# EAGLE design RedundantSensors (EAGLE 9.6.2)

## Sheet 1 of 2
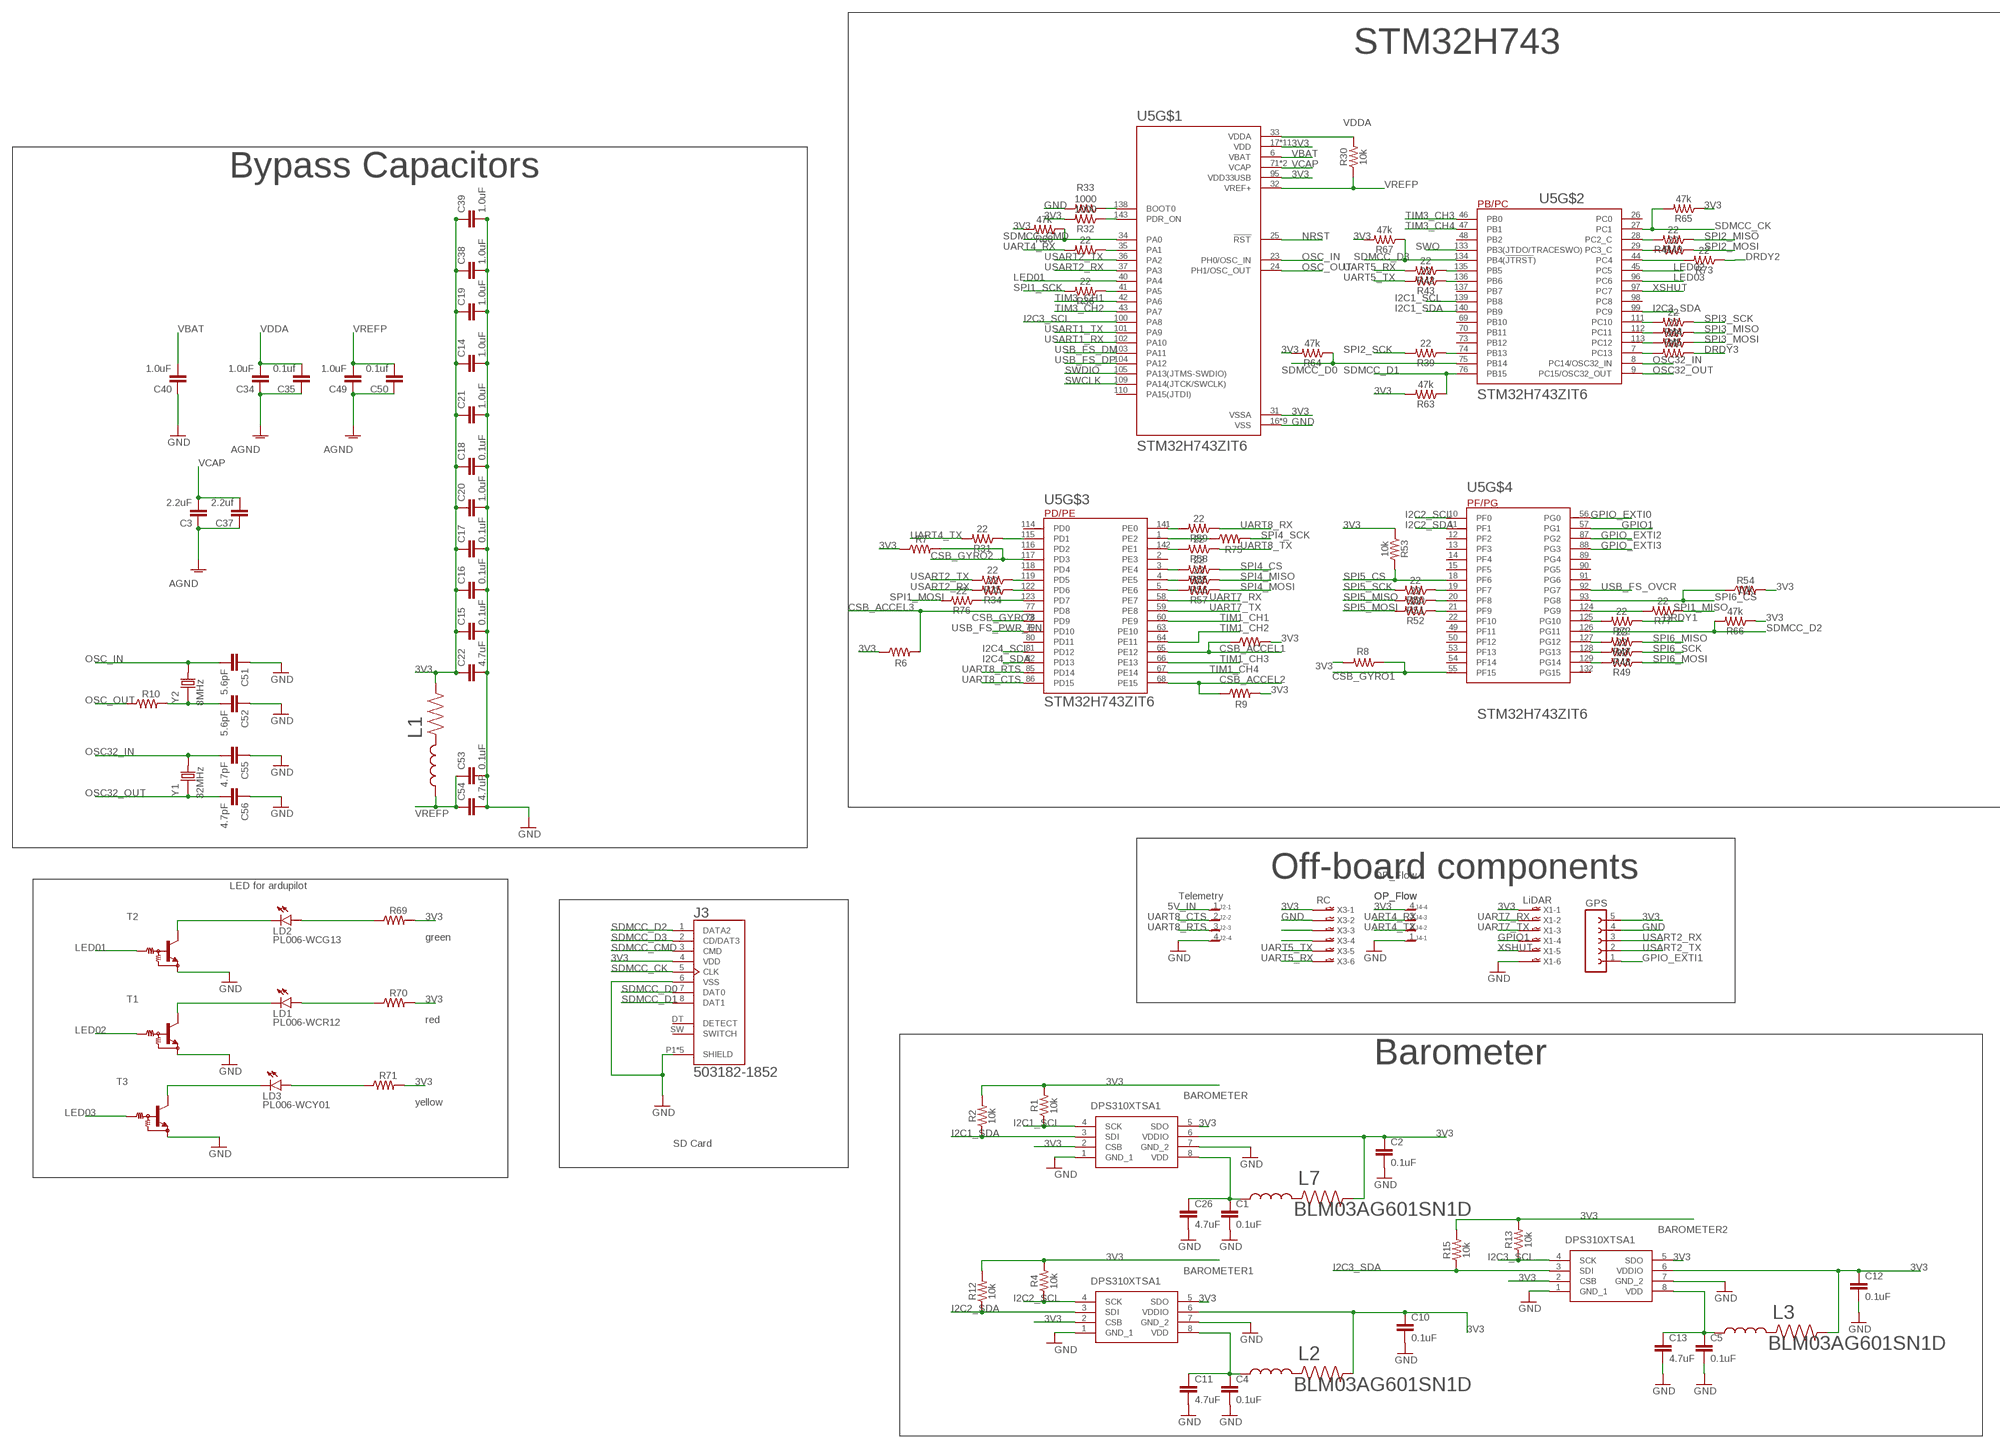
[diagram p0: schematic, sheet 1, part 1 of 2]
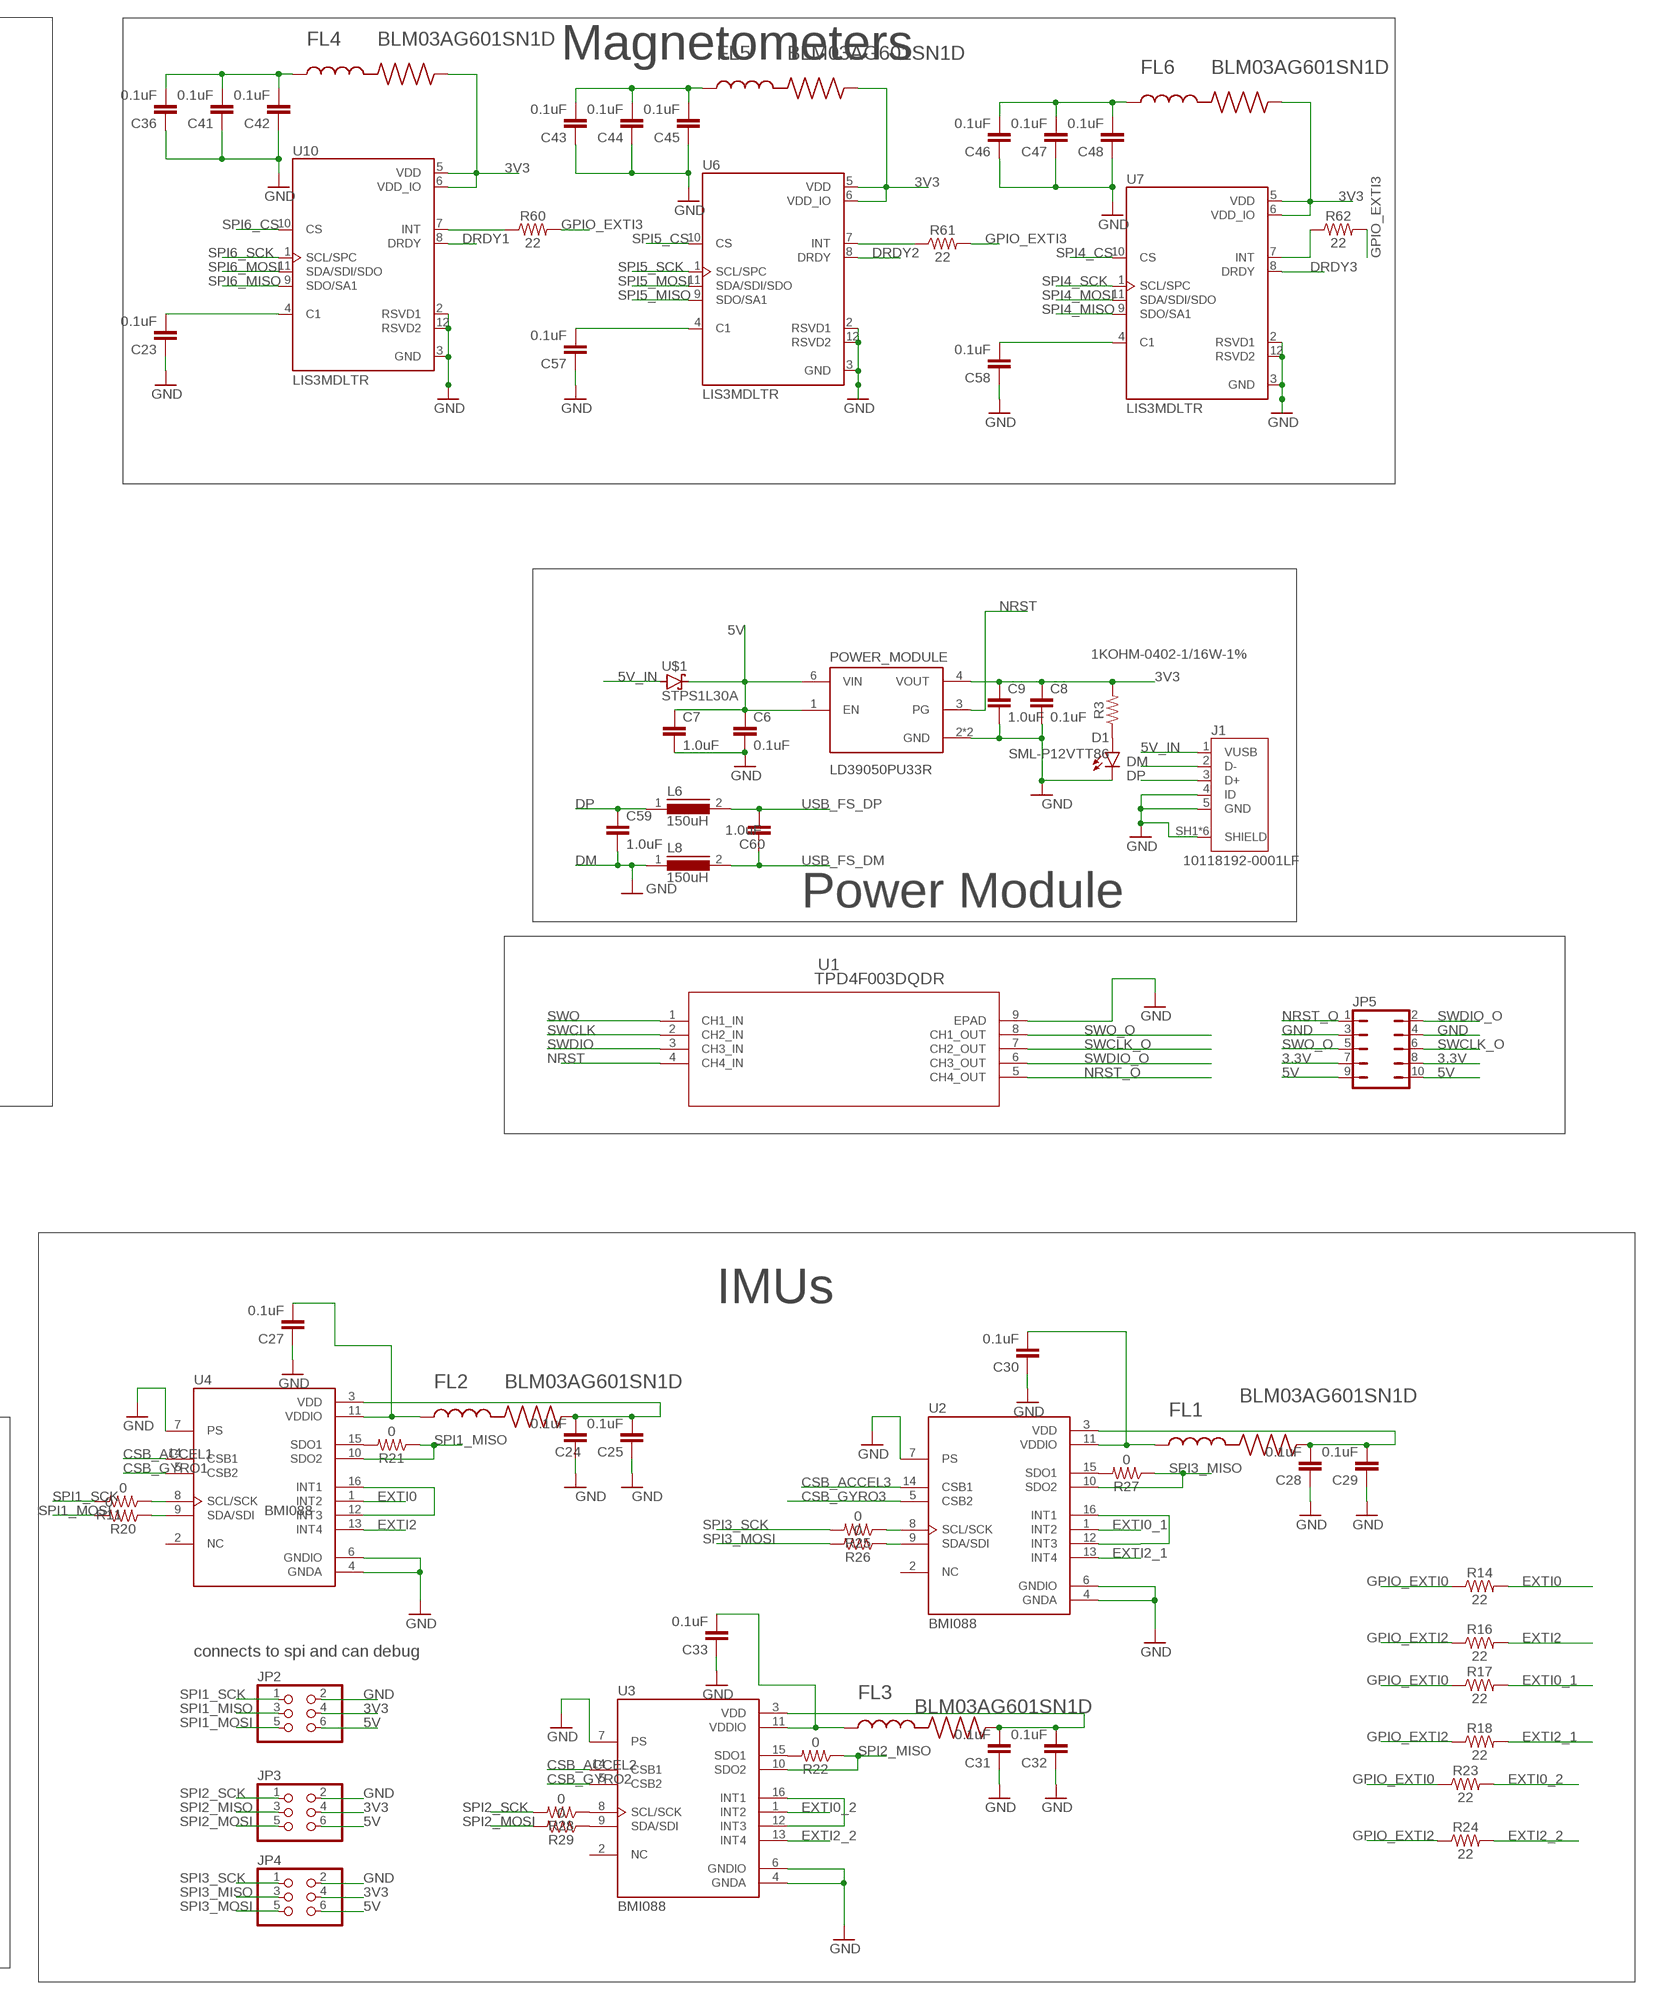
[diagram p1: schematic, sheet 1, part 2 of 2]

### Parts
BAROMETER  DPS310XTSA1  [DPS310XTSA1]
BAROMETER1  DPS310XTSA1  [DPS310XTSA1]
BAROMETER2  DPS310XTSA1  [DPS310XTSA1]
C1  0.1uF  0.1UF-0402-6.3V-10%-X7R  [0402]
C2  0.1uF  0.1UF-0402-6.3V-10%-X7R  [0402]
C3  2.2uF  1.0UF-0805-25V-10%  [0805]
C4  0.1uF  0.1UF-0402-6.3V-10%-X7R  [0402]
C5  0.1uF  0.1UF-0402-6.3V-10%-X7R  [0402]
C6  0.1uF  0.1UF-0402-6.3V-10%-X7R  [0402]
C7  1.0uF  1.0UF-0402-16V-10%  [0402]
C8  0.1uF  0.1UF-0402-6.3V-10%-X7R  [0402]
C9  1.0uF  1.0UF-0402-16V-10%  [0402]
C10  0.1uF  0.1UF-0402-6.3V-10%-X7R  [0402]
C11  4.7uF  4.7UF0603  [0603]
C12  0.1uF  0.1UF-0402-6.3V-10%-X7R  [0402]
C13  4.7uF  4.7UF0603  [0603]
C14  1.0uF  1.0UF-0805-25V-10%  [0805]
C15  0.1uF  0.1UF-0603-25V-5%  [0603]
C16  0.1uF  0.1UF-0603-25V-5%  [0603]
C17  0.1uF  0.1UF-0603-25V-5%  [0603]
C18  0.1uF  0.1UF-0603-25V-5%  [0603]
C19  1.0uF  1.0UF-0805-25V-10%  [0805]
C20  1.0uF  1.0UF-0805-25V-10%  [0805]
C21  1.0uF  1.0UF-0805-25V-10%  [0805]
C22  4.7uF  4.7UF0603  [0603]
C23  0.1uF  0.1UF-0603-25V-5%  [0603]
C24  0.1uF  0.1UF-0603-25V-5%  [0603]
C25  0.1uF  0.1UF-0603-25V-5%  [0603]
C26  4.7uF  4.7UF0603  [0603]
C27  0.1uF  0.1UF-0603-25V-5%  [0603]
C28  0.1uF  0.1UF-0603-25V-5%  [0603]
C29  0.1uF  0.1UF-0603-25V-5%  [0603]
C30  0.1uF  0.1UF-0603-25V-5%  [0603]
C31  0.1uF  0.1UF-0603-25V-5%  [0603]
C32  0.1uF  0.1UF-0603-25V-5%  [0603]
C33  0.1uF  0.1UF-0603-25V-5%  [0603]
C34  1.0uF  1.0UF-0805-25V-10%  [0805]
C35  0.1uf  1.0UF-0805-25V-10%  [0805]
C36  0.1uF  0.1UF-0603-25V-5%  [0603]
C37  2.2uf  1.0UF-0805-25V-10%  [0805]
C38  1.0uF  1.0UF-0805-25V-10%  [0805]
C39  1.0uF  1.0UF-0805-25V-10%  [0805]
C40  1.0uF  1.0UF-0805-25V-10%  [0805]
C41  0.1uF  0.1UF-0603-25V-5%  [0603]
C42  0.1uF  0.1UF-0603-25V-5%  [0603]
C43  0.1uF  0.1UF-0603-25V-5%  [0603]
C44  0.1uF  0.1UF-0603-25V-5%  [0603]
C45  0.1uF  0.1UF-0603-25V-5%  [0603]
C46  0.1uF  0.1UF-0603-25V-5%  [0603]
C47  0.1uF  0.1UF-0603-25V-5%  [0603]
C48  0.1uF  0.1UF-0603-25V-5%  [0603]
C49  1.0uF  1.0UF-0805-25V-10%  [0805]
C50  0.1uf  1.0UF-0805-25V-10%  [0805]
C51  5.6pF  1.0UF-0805-25V-10%  [0805]
C52  5.6pF  1.0UF-0805-25V-10%  [0805]
C53  0.1uF  0.1UF-0603-25V-5%  [0603]
C54  4.7uF  4.7UF0603  [0603]
C55  4.7pF  1.0UF-0805-25V-10%  [0805]
C56  4.7pF  1.0UF-0805-25V-10%  [0805]
C57  0.1uF  0.1UF-0603-25V-5%  [0603]
C58  0.1uF  0.1UF-0603-25V-5%  [0603]
C59  1.0uF  1.0UF-0402-16V-10%  [0402]
C60  1.0uF  1.0UF-0402-16V-10%  [0402]
D1  SML-P12VTT86  [LED_SML-P11UTT86R]
FL1  BLM03AG601SN1D  [BEADC0603X33N]
FL2  BLM03AG601SN1D  [BEADC0603X33N]
FL3  BLM03AG601SN1D  [BEADC0603X33N]
FL4  BLM03AG601SN1D  [BEADC0603X33N]
FL5  BLM03AG601SN1D  [BEADC0603X33N]
FL6  BLM03AG601SN1D  [BEADC0603X33N]
GPS  FE05-1  [FE05-1]
J1  10118192-0001LF  [AMPHENOL_10118192-0001LF]
J2  JST-SH-4_SMT_V  [BM04B-SRSS-TB]
J3  503182-1852  [MOLEX_503182-1852]
J4  JST-SH-4_SMT_V  [BM04B-SRSS-TB]
JP2  PINHD-2X3  [2X03]
JP3  PINHD-2X3  [2X03]
JP4  PINHD-2X3  [2X03]
JP5  JP5Q  [JP5Q]
L1  BLM03AG601SN1D  [BEADC0603X33N]
L2  BLM03AG601SN1D  [BEADC0603X33N]
L3  BLM03AG601SN1D  [BEADC0603X33N]
L6  150uH  MICC10  [MICC10]
L7  BLM03AG601SN1D  [BEADC0603X33N]
L8  150uH  MICC10  [MICC10]
LD1  PL006-WCR12  [SOT23]
LD2  PL006-WCG13  PL006-WCR12  [SOT23]
LD3  PL006-WCY01  PL006-WCR12  [SOT23]
POWER_MODULE  LD39050PU33R  [SON95P300X300X100-7N]
R1  10k  10KOHM-0402-1/16W-1%  [0402]
R2  10k  10KOHM-0402-1/16W-1%  [0402]
R3  1KOHM-0402-1/16W-1%  [0402]
R4  10k  10KOHM-0402-1/16W-1%  [0402]
R5  22  10KOHM-0402-1/16W-1%  [0402]
R6  10k  RT0402FRE07220RL  [RESC1005X35N]
R7  10k  RT0402FRE07220RL  [RESC1005X35N]
R8  10k  RT0402FRE07220RL  [RESC1005X35N]
R9  10k  RT0402FRE07220RL  [RESC1005X35N]
R10  220  RT0402FRE07220RL  [RESC1005X35N]
R11  0  10KOHM-0402-1/16W-1%  [0402]
R12  10k  10KOHM-0402-1/16W-1%  [0402]
R13  10k  10KOHM-0402-1/16W-1%  [0402]
R14  22  22OHM-0402-1/10W-1%  [0402]
R15  10k  10KOHM-0402-1/16W-1%  [0402]
R16  22  22OHM-0402-1/10W-1%  [0402]
R17  22  22OHM-0402-1/10W-1%  [0402]
R18  22  22OHM-0402-1/10W-1%  [0402]
R19  10k  RT0402FRE07220RL  [RESC1005X35N]
R20  0  10KOHM-0402-1/16W-1%  [0402]
R21  0  10KOHM-0402-1/16W-1%  [0402]
R22  0  10KOHM-0402-1/16W-1%  [0402]
R23  22  22OHM-0402-1/10W-1%  [0402]
R24  22  22OHM-0402-1/10W-1%  [0402]
R25  0  10KOHM-0402-1/16W-1%  [0402]
R26  0  10KOHM-0402-1/16W-1%  [0402]
R27  0  10KOHM-0402-1/16W-1%  [0402]
R28  0  10KOHM-0402-1/16W-1%  [0402]
R29  0  10KOHM-0402-1/16W-1%  [0402]
R30  10k  10KOHM-0402-1/16W-1%  [0402]
R31  22  10KOHM-0402-1/16W-1%  [0402]
R32  1000  10KOHM-0402-1/16W-1%  [0402]
R33  1000  10KOHM-0402-1/16W-1%  [0402]
R34  22  10KOHM-0402-1/16W-1%  [0402]
R35  22  10KOHM-0402-1/16W-1%  [0402]
R36  22  10KOHM-0402-1/16W-1%  [0402]
R39  22  10KOHM-0402-1/16W-1%  [0402]
R40  22  10KOHM-0402-1/16W-1%  [0402]
R41  22  10KOHM-0402-1/16W-1%  [0402]
R42  22  10KOHM-0402-1/16W-1%  [0402]
R43  22  10KOHM-0402-1/16W-1%  [0402]
R44  22  10KOHM-0402-1/16W-1%  [0402]
R45  22  10KOHM-0402-1/16W-1%  [0402]
R46  22  10KOHM-0402-1/16W-1%  [0402]
R47  22  10KOHM-0402-1/16W-1%  [0402]
R48  22  10KOHM-0402-1/16W-1%  [0402]
R49  22  10KOHM-0402-1/16W-1%  [0402]
R50  22  10KOHM-0402-1/16W-1%  [0402]
R51  22  10KOHM-0402-1/16W-1%  [0402]
R52  22  10KOHM-0402-1/16W-1%  [0402]
R53  10k  10KOHM-0402-1/16W-1%  [0402]
R54  10k  10KOHM-0402-1/16W-1%  [0402]
R55  22  10KOHM-0402-1/16W-1%  [0402]
R56  22  10KOHM-0402-1/16W-1%  [0402]
R57  22  10KOHM-0402-1/16W-1%  [0402]
R58  22  10KOHM-0402-1/16W-1%  [0402]
R59  22  10KOHM-0402-1/16W-1%  [0402]
R60  22  22OHM-0402-1/10W-1%  [0402]
R61  22  22OHM-0402-1/10W-1%  [0402]
R62  22  22OHM-0402-1/10W-1%  [0402]
R63  47k  10KOHM-0402-1/16W-1%  [0402]
R64  47k  10KOHM-0402-1/16W-1%  [0402]
R65  47k  10KOHM-0402-1/16W-1%  [0402]
R66  47k  10KOHM-0402-1/16W-1%  [0402]
R67  47k  10KOHM-0402-1/16W-1%  [0402]
R68  47k  10KOHM-0402-1/16W-1%  [0402]
R69  270  RT0402FRE07220RL  [RESC1005X35N]
R70  270  RT0402FRE07220RL  [RESC1005X35N]
R71  270  RT0402FRE07220RL  [RESC1005X35N]
R72  22  10KOHM-0402-1/16W-1%  [0402]
R73  22  10KOHM-0402-1/16W-1%  [0402]
R74  22  10KOHM-0402-1/16W-1%  [0402]
R75  10k  RT0402FRE07220RL  [RESC1005X35N]
R76  22  10KOHM-0402-1/16W-1%  [0402]
R77  22  10KOHM-0402-1/16W-1%  [0402]
T1  MUN2213T1-NPN_DRIVER-SC59-BEC  [SC59-BEC]
T2  MUN2213T1-NPN_DRIVER-SC59-BEC  [SC59-BEC]
T3  MUN2213T1-NPN_DRIVER-SC59-BEC  [SC59-BEC]
U1  TPD4F003DQDR  [DQD8_1P2X0P4]
U2  BMI088  [PQFN50P450X300X100-16N]
U3  BMI088  [PQFN50P450X300X100-16N]
U4  BMI088  [PQFN50P450X300X100-16N]
U5  STM32H743ZIT6  [QFP50P2200X2200X160-144N]
U6  LIS3MDLTR  [XDCR_LIS3MDLTR]
U7  LIS3MDLTR  [XDCR_LIS3MDLTR]
U10  LIS3MDLTR  [XDCR_LIS3MDLTR]
U$1  STPS1L30A  [DIOM5226X223N]
X1  LiDAR  06FLZ-SM1  [6FLZ-SM]
X3  RC  06FLZ-SM1  [6FLZ-SM]
Y1  32MHz  ABLS-8.000MHZ-B2-T  [XTAL_ABLS-8.000MHZ-B2-T]
Y2  8MHz  ABLS-8.000MHZ-B2-T  [XTAL_ABLS-8.000MHZ-B2-T]

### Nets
3.3V: JP5.7 JP5.8
3V2: C28.2 C29.2 FL1.2 U2.3(VDD)
3V3: BAROMETER1.2(CSB) BAROMETER1.5(SDO) BAROMETER1.6(VDDIO) BAROMETER2.2(CSB) BAROMETER2.5(SDO) BAROMETER2.6(VDDIO) BAROMETER.2(CSB) BAROMETER.5(SDO) BAROMETER.6(VDDIO) C2.1 C8.1 C9.1 C10.1 C12.1 C14.1 C15.1 C16.1 C17.1 C18.1 C19.1 C20.1 C21.1 C22.1 C38.1 C39.1 FL4.2 FL5.2 FL6.2 GPS.5 J3.4(VDD) J4.4 JP2.4 JP3.4 JP4.4 L1.2 L2.2 L3.2 L7.2 POWER_MODULE.4(VOUT) R1.2 R2.2 R3.2 R4.2 R6.1 R7.1 R8.2 R9.2 R12.2 R13.2 R15.2 R19.2 R32.2 R53.1 R54.2 R63.2 R64.2 R65.1 R66.1 R67.2 R68.2 R69.2 R70.2 R71.2 U5.17(VDD) U5.30(VDD) U5.31(VSSA) U5.39(VDD) U5.52(VDD) U5.62(VDD) U5.72(VDD) U5.84(VDD) U5.95(VDD33USB) U5.108(VDD) U5.121(VDD) U5.131(VDD) U5.144(VDD) U6.5(VDD) U6.6(VDD_IO) U7.5(VDD) U7.6(VDD_IO) U10.5(VDD) U10.6(VDD_IO) X1.1 X3.1
3V4: C24.2 C25.2 FL2.2 U4.3(VDD)
3V5: C31.2 C32.2 FL3.2 U3.3(VDD)
5V: C6.1 C7.1 JP2.6 JP3.6 JP4.6 JP5.9 JP5.10 POWER_MODULE.1(EN) POWER_MODULE.6(VIN) U$1.1(C)
5V_IN: J1.1(VUSB) J2.1 U$1.2(A)
AGND: C3.1 C34.1 C35.1 C37.1 C49.1 C50.1
CSB_ACCEL1: R19.1 U4.14(CSB1) U5.65(PE12)
CSB_ACCEL2: R9.1 U3.14(CSB1) U5.68(PE15)
CSB_ACCEL3: R6.2 U2.14(CSB1) U5.77(PD8)
CSB_GYRO1: R8.1 U4.5(CSB2) U5.55(PF15)
CSB_GYRO2: R7.2 U3.5(CSB2) U5.117(PD3)
CSB_GYRO3: U2.5(CSB2) U5.78(PD9)
DM: C59.2 J1.2(D-) L8.1 ; supply symbol labelled GND
DP: C59.1 J1.3(D+) L6.1
DRDY1: R72.1 U10.8(DRDY)
DRDY2: R73.1 R73.2 U5.44(PC4) U6.8(DRDY)
DRDY3: R74.1 U7.8(DRDY)
EXTI0: R14.2 U4.1(INT2)
EXTI0_1: R17.2 U2.1(INT2)
EXTI0_2: R23.2 U3.1(INT2)
EXTI2: R16.2 U4.13(INT4)
EXTI2_1: R18.2 U2.13(INT4)
EXTI2_2: R24.2 U3.13(INT4)
GND: BAROMETER1.1(GND_1) BAROMETER1.7(GND_2) BAROMETER2.1(GND_1) BAROMETER2.7(GND_2) BAROMETER.1(GND_1) BAROMETER.7(GND_2) C1.2 C2.2 C4.2 C5.2 C6.2 C7.2 C8.2 C9.2 C10.2 C11.2 C12.2 C13.2 C14.2 C15.2 C16.2 C17.2 C18.2 C19.2 C20.2 C21.2 C22.2 C23.1 C24.1 C25.1 C26.2 C27.1 C28.1 C29.1 C30.1 C31.1 C32.1 C33.1 C36.1 C38.2 C39.2 C40.1 C41.1 C42.1 C43.1 C44.1 C45.1 C46.1 C47.1 C48.1 C51.1 C52.1 C53.2 C54.2 C55.1 C56.1 C57.1 C58.1 D1.C GPS.4 J1.4(ID) J1.5(GND) J1.SH1(SHIELD) J1.SH2(SHIELD) J1.SH3(SHIELD) J1.SH4(SHIELD) J1.SH5(SHIELD) J1.SH6(SHIELD) J3.6(VSS) J3.P1(SHIELD) J3.P2(SHIELD) J3.P3(SHIELD) J3.P4(SHIELD) J3.P5(SHIELD) J4.1 JP2.2 JP3.2 JP4.2 JP5.3 JP5.4 POWER_MODULE.2(GND) POWER_MODULE.7(GND) R33.2 T1.E T2.E T3.E U1.9(EPAD) U2.4(GNDA) U2.6(GNDIO) U2.7(PS) U3.4(GNDA) U3.6(GNDIO) U3.7(PS) U4.4(GNDA) U4.6(GNDIO) U4.7(PS) U5.16(VSS) U5.38(VSS) U5.51(VSS) U5.61(VSS) U5.83(VSS) U5.94(VSS) U5.107(VSS) U5.120(VSS) U5.130(VSS) U6.2(RSVD1) U6.3(GND) U6.12(RSVD2) U7.2(RSVD1) U7.3(GND) U7.12(RSVD2) U10.2(RSVD1) U10.3(GND) U10.12(RSVD2) X1.6 X3.2
GPIO1: U5.57(PG1) X1.4
GPIO_EXTI0: R14.1 R17.1 R23.1 U5.56(PG0)
GPIO_EXTI1: GPS.1
GPIO_EXTI2: R16.1 R18.1 R24.1 U5.87(PG2)
GPIO_EXTI3: R60.2 R61.2 R62.2 U5.88(PG3)
I2C1_SCL: BAROMETER.4(SCK) R1.1 U5.139(PB8)
I2C1_SDA: BAROMETER.3(SDI) R2.1 U5.140(PB9)
I2C2_SCL: BAROMETER1.4(SCK) R4.1 U5.10(PF0)
I2C2_SDA: BAROMETER1.3(SDI) R12.1 U5.11(PF1)
I2C3_SCL: BAROMETER2.4(SCK) R13.1 U5.100(PA8)
I2C3_SDA: BAROMETER2.3(SDI) R15.1 U5.99(PC9)
I2C4_SCL: U5.81(PD12)
I2C4_SDA: U5.82(PD13)
INT1: U2.12(INT3) U2.16(INT1)
LED01: T2.B U5.40(PA4)
LED02: T1.B U5.45(PC5)
LED03: T3.B U5.96(PC6)
N$1: U4.12(INT3) U4.16(INT1)
N$2: BAROMETER2.8(VDD) C5.1 C13.1 L3.1
N$3: BAROMETER1.8(VDD) C4.1 C11.1 L2.1
N$4: U3.12(INT3) U3.16(INT1)
N$5: D1.A R3.1
N$6: BAROMETER.8(VDD) C1.1 C26.1 L7.1
N$7: C52.2 R10.2 Y2.1
N$8: C27.2 FL2.1 U4.11(VDDIO)
N$9: C30.2 FL1.1 U2.11(VDDIO)
N$10: C33.2 FL3.1 U3.11(VDDIO)
N$11: C23.2 U10.4(C1)
N$12: R32.1 U5.143(PDR_ON)
N$13: R55.2 U5.3(PE4)
N$14: R56.2 U5.4(PE5)
N$15: X3.4
N$16: C36.2 C41.2 C42.2 FL4.1
N$17: C57.2 U6.4(C1)
N$18: R33.1 U5.138(BOOT0)
N$19: J2.4 ; supply symbol labelled GND
N$20: R5.1 U5.35(PA1)
N$21: R11.1 U4.8(SCL/SCK)
N$22: R20.1 U4.9(SDA/SDI)
N$23: R40.2 U5.28(PC2_C)
N$24: R21.2 U4.15(SDO1)
N$25: R22.2 U3.15(SDO1)
N$26: R25.1 U2.8(SCL/SCK)
N$27: R26.1 U2.9(SDA/SDI)
N$28: R27.2 U2.15(SDO1)
N$29: R28.1 U3.8(SCL/SCK)
N$30: R29.1 U3.9(SDA/SDI)
N$31: R34.1 U5.122(PD6)
N$32: R35.1 U5.119(PD5)
N$33: R36.1 U5.41(PA5)
N$36: R39.1 U5.74(PB13)
N$37: R41.2 U5.29(PC3_C)
N$38: R31.1 U5.115(PD1)
N$39: R42.1 U5.135(PB5)
N$40: R43.1 U5.136(PB6)
N$41: R44.2 U5.111(PC10)
N$42: R45.2 U5.112(PC11)
N$43: R46.2 U5.113(PC12)
N$44: R47.2 U5.127(PG12)
N$45: R48.2 U5.128(PG13)
N$46: R49.2 U5.129(PG14)
N$47: R50.1 U5.19(PF7)
N$48: R51.1 U5.20(PF8)
N$49: R52.1 U5.21(PF9)
N$50: R57.2 U5.5(PE6)
N$51: R58.2 U5.142(PE1)
N$52: R59.2 U5.141(PE0)
N$53: C43.2 C44.2 C45.2 FL5.1
N$54: C58.2 U7.4(C1)
N$55: C46.2 C47.2 C48.2 FL6.1
N$56: R60.1 U10.7(INT)
N$57: R61.1 U6.7(INT)
N$58: R62.1 U7.7(INT)
N$59: LD2.3(C) T2.C
N$60: LD2.1(A) R69.1
N$61: LD1.3(C) T1.C
N$62: LD1.1(A) R70.1
N$63: LD3.3(C) T3.C
N$64: LD3.1(A) R71.1
N$65: R72.2 U5.125(PG10)
N$66: R74.2 U5.7(PC13)
N$67: R75.1 U5.1(PE2)
N$68: R76.1 U5.123(PD7)
N$69: R77.2 U5.124(PG9)
NRST: POWER_MODULE.3(PG) U1.4(CH4_IN) U5.25(!RST)
NRST_O: JP5.1 U1.5(CH4_OUT)
OSC32_IN: C55.2 U5.8(PC14/OSC32_IN) Y1.2
OSC32_OUT: C56.2 U5.9(PC15/OSC32_OUT) Y1.1
OSC_IN: C51.2 U5.23(PH0/OSC_IN) Y2.2
OSC_OUT: R10.1 U5.24(PH1/OSC_OUT)
SDMCC_CK: J3.5(CLK) R65.2 U5.27(PC1)
SDMCC_CMD: J3.3(CMD) R68.1 U5.34(PA0)
SDMCC_D0: J3.7(DAT0) R64.1 U5.75(PB14)
SDMCC_D1: J3.8(DAT1) R63.1 U5.76(PB15)
SDMCC_D2: J3.1(DATA2) R66.2 U5.126(PG11)
SDMCC_D3: J3.2(CD/DAT3) R67.1 U5.134(PB4(!JTRST!))
SPI1_MISO: JP2.3 R21.1 R77.1 U4.10(SDO2)
SPI1_MOSI: JP2.5 R20.2 R76.2
SPI1_SCK: JP2.1 R11.2 R36.2
SPI2_MISO: JP3.3 R22.1 R40.1 U3.10(SDO2)
SPI2_MOSI: JP3.5 R29.2 R41.1
SPI2_SCK: JP3.1 R28.2 R39.2
SPI3_MISO: JP4.3 R27.1 R45.1 U2.10(SDO2)
SPI3_MOSI: JP4.5 R26.2 R46.1
SPI3_SCK: JP4.1 R25.2 R44.1
SPI4_CS: R55.1 U7.10(CS)
SPI4_MISO: R56.1 U7.9(SDO/SA1)
SPI4_MOSI: R57.1 U7.11(SDA/SDI/SDO)
SPI4_SCK: R75.2 U7.1(SCL/SPC)
SPI5_CS: R53.2 U5.18(PF6) U6.10(CS)
SPI5_MISO: R51.2 U6.9(SDO/SA1)
SPI5_MOSI: R52.2 U6.11(SDA/SDI/SDO)
SPI5_SCK: R50.2 U6.1(SCL/SPC)
SPI6_CS: R54.1 U5.93(PG8) U10.10(CS)
SPI6_MISO: R47.1 U10.9(SDO/SA1)
SPI6_MOSI: R49.1 U10.11(SDA/SDI/SDO)
SPI6_SCK: R48.1 U10.1(SCL/SPC)
SWCLK: U1.2(CH2_IN) U5.109(PA14(JTCK/SWCLK))
SWCLK_O: JP5.6 U1.7(CH2_OUT)
SWDIO: U1.3(CH3_IN) U5.105(PA13(JTMS-SWDIO))
SWDIO_O: JP5.2 U1.6(CH3_OUT)
SWO: U1.1(CH1_IN) U5.133(PB3(JTDO/TRACESWO))
SWO_O: JP5.5 U1.8(CH1_OUT)
TIM1_CH1: U5.60(PE9)
TIM1_CH2: U5.64(PE11)
TIM1_CH3: U5.66(PE13)
TIM1_CH4: U5.67(PE14)
TIM3_CH1: U5.42(PA6)
TIM3_CH2: U5.43(PA7)
TIM3_CH3: U5.46(PB0)
TIM3_CH4: U5.47(PB1)
UART4_RX: J4.3 R5.2
UART4_TX: J4.2 R31.2
UART5_RX: R42.2 X3.3 X3.6
UART5_TX: R43.2 X3.5
UART7_RX: U5.58(PE7) X1.2
UART7_TX: U5.59(PE8) X1.3
UART8_CTS: J2.2 U5.86(PD15)
UART8_RTS: J2.3 U5.85(PD14)
UART8_RX: R59.1
UART8_TX: R58.1
USART1_RX: U5.102(PA10)
USART1_TX: U5.101(PA9)
USART2_RX: GPS.3 R34.2 U5.37(PA3)
USART2_TX: GPS.2 R35.2 U5.36(PA2)
USB_FS_DM: C60.2 L8.2 U5.103(PA11)
USB_FS_DP: C60.1 L6.2 U5.104(PA12)
USB_FS_OVCR: U5.92(PG7)
USB_FS_PWR_EN: U5.79(PD10)
VBAT: C40.2 U5.6(VBAT)
VCAP: C3.2 C37.2 U5.71(VCAP) U5.106(VCAP)
VDDA: C34.2 C35.2 R30.2 U5.33(VDDA)
VREFP: C49.2 C50.2 C53.1 C54.1 L1.1 R30.1 U5.32(VREF+)
XSHUT: U5.97(PC7) X1.5
Unconnected: J2.M1 J2.M2 J3.DT(DETECT) J3.SW(SWITCH) J4.M1 J4.M2 U2.2(NC) U3.2(NC) U4.2(NC) U5.2(PE3) U5.12(PF2) U5.13(PF3) U5.14(PF4) U5.15(PF5) U5.22(PF10) U5.26(PC0) U5.48(PB2) U5.49(PF11) U5.50(PF12) U5.53(PF13) U5.54(PF14) U5.63(PE10) U5.69(PB10) U5.70(PB11) U5.73(PB12) U5.80(PD11) U5.89(PG4) U5.90(PG5) U5.91(PG6) U5.98(PC8) U5.110(PA15(JTDI)) U5.114(PD0) U5.116(PD2) U5.118(PD4) U5.132(PG15) U5.137(PB7)

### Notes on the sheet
- STM32H743 | Magnetometers
- Bypass Capacitors
- Power Module
- Off-board components | OP_Flow
- LED for ardupilot
- Telemetry | OP_Flow | OP_Flow
- green
- IMUs
- red
- Barometer
- yellow
- SD Card
- connects to spi and can debug

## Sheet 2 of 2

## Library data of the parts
BAROMETER BAROMETER1 BAROMETER2 = DPS310XTSA1:DPS310XTSA1: INFINEON - DPS310XTSA1 - DIGITAL PRESSURE SENSOR, 1200HPA, VLGA-8 Source: Datasheet; ARROW_PART_NUMBER: DPS310XTSA1; ARROW_PRICE-STOCK: https://www.arrow.com/en/products/dps310xtsa1/infineon-technologies-ag?region=nac; DESCRIPTION: INFINEON - DPS310XTSA1 - DIGITAL PRESSURE SENSOR, 1200HPA, VLGA-8; HEIGHT: 1.01mm; MANUFACTURER_NAME: Infineon; MANUFACTURER_PART_NUMBER: DPS310XTSA1; MOUSER_PART_NUMBER: 726-DPS310XTSA1; MOUSER_PRICE-STOCK: https://www.mouser.co.uk/ProductDetail/Infineon-Technologies/DPS310XTSA1?qs=uuTTuBTXn66Ynca8WHwycg%3D%3D
C1 C2 C4-C6 C8 C10 C12 = SparkFun-Capacitors:0.1UF: 0.1µF ceramic capacitors; PROD_ID: CAP-14993
C3 C35 C37 C50-C52 C55 C56 = SparkFun-Capacitors:1.0UF: 1µF ceramic capacitors; PROD_ID: CAP-08064; VALUE: 1.0uF
C7 C9 C59 C60 = SparkFun-Capacitors:1.0UF: 1µF ceramic capacitors; PROD_ID: CAP-12417
C11 C13 C22 C26 C54 = SparkFun-Capacitors:4.7UF: 4.7µF ceramic capacitors; PROD_ID: CAP-08280
C14 C19-C21 C34 C38-C40 C49 = SparkFun-Capacitors:1.0UF: 1µF ceramic capacitors; PROD_ID: CAP-08064
C15-C18 C23-C25 C27-C33 C36 C41-C48 C53 C57 C58 = SparkFun-Capacitors:0.1UF: 0.1µF ceramic capacitors; PROD_ID: CAP-08604
D1 = ce-capstone:SML-P12VTT86: SML-P1 Series Red 0402 Clear 60 mcd 2 V Surface Mount PICOLED LED; AVAILABILITY: Unavailable; DESCRIPTION: Red 630nm LED Indication - Discrete 2V 0402 _1006 Metric_; MF: Rohm; MP: SML-P12VTT86; PACKAGE: 0402 Rohm; PRICE: None
FL1-FL6 L1-L3 L7 = BLM03AG601SN1D:BLM03AG601SN1D: Ferrite Bead 600R 100mA SMD 0201 Check availability; AVAILABILITY: In Stock; CHECK_PRICES: https://www.snapeda.com/parts/BLM03AG601SN1D/Murata/view-part/?ref=eda; DESCRIPTION: 600 Ohms @ 100 MHz 1 - Ferrite Bead 0201 (0603 Metric) 100mA 1.5Ohm; MF: Murata Electronics; MP: BLM03AG601SN1D; PACKAGE: 0603 Murata; PRICE: None; PURCHASE-URL: https://www.snapeda.com/api/url_track_click_mouser/?unipart_id=283112&manufacturer=Murata Electronics&part_name=BLM03AG601SN1D&search_term=None; SNAPEDA_LINK: https://www.snapeda.com/parts/BLM03AG601SN1D/Murata/view-part/?ref=snap
GPS = con-lsta:FE05-1: FEMALE HEADER; OC_FARNELL: unknown; OC_NEWARK: unknown
J1 = ce-capstone:10118192-0001LF: Single Port 5 Contact Horizontal Right Angle Shielded Micro B USB 2.0 Connector; AVAILABILITY: Unavailable; DESCRIPTION: USB - micro B USB 2.0 Receptacle Connector 5 Position Surface Mount, Right Angle; MF: Amphenol ICC; MP: 10118192-0001LF; PACKAGE: None; PRICE: None
J2 J4 = con-JST-SH:JST-SH-4; MF: JST; MPN: BM04B-SRSS-TB
J3 = 503182-1852:503182-1852: Conn Micro SD Card M 8 POS 1.09mm Solder RA SMD Embossed T/R 0.5A/Contact Check availability; AVAILABILITY: In Stock; CHECK_PRICES: https://www.snapeda.com/parts/5031821852/Molex/view-part/?ref=eda; DESCRIPTION: 10 (8 + 2) Position Card Connector Secure Digital - microSD™ Surface Mount, Right Angle Gold; MF: Molex; MP: 5031821852; PACKAGE: None; PRICE: None; PURCHASE-URL: https://www.snapeda.com/api/url_track_click_mouser/?unipart_id=46835&manufacturer=Molex&part_name=5031821852&search_term=None; SNAPEDA_LINK: https://www.snapeda.com/parts/5031821852/Molex/view-part/?ref=snap
JP2-JP4 = pinhead:PINHD-2X3: PIN HEADER
JP5 = jumper:JP5Q: JUMPER
L6 L8 = inductors:MICC10: INDUCTOR; SPICEPREFIX: L
LD1-LD3 = led:PL006*: PLH006 Series SMD LED SOT23
POWER_MODULE = ce-capstone:LD39050PU33R: LD39050 Series 500 mA 3.3 V Fixed Low Noise LDO Voltage Regulator - DFN-6; AVAILABILITY: Unavailable; DESCRIPTION: Linear Voltage Regulator IC 1 Output 500mA 6-DFN _3x3_; MF: STMicroelectronics; MP: LD39050PU33R; PACKAGE: DFN-6 STMicroelectronics; PRICE: None
R1 R2 R4 R12 R13 R15 R30 R53 R54 = SparkFun-Resistors:10KOHM: 10kΩ resistor; PROD_ID: RES-14241
R3 = SparkFun-Resistors:1KOHM: 1kΩ resistor; PROD_ID: RES-14342
R5 R11 R20-R22 R25-R29 R31-R36 R39-R52 R55-R59 R63-R68 R72-R74 R76 R77 = SparkFun-Resistors:10KOHM: 10kΩ resistor; PROD_ID: RES-14241; VALUE: 10k
R6-R10 R19 R69-R71 R75 = ce-capstone:RT0402FRE07220RL: RES SMD 4.7K OHM 1% 1/16W 0402; DESCRIPTION: 4.7 kOhms ±1% 0.063W, 1/16W Chip Resistor 0402 _1005 Metric_ Thin Film; DIGI-KEY_PART_NUMBER: YAG3347CT-ND; DIGI-KEY_PURCHASE_URL: https://www.digikey.com/product-detail/en/yageo/RT0402FRE074K7L/YAG3347CT-ND/5418052?utm_source=snapeda&utm_medium=aggregator&utm_campaign=symbol; MF: Yageo; MP: RT0402FRE074K7L; PACKAGE: 1005 Yageo
R14 R16-R18 R23 R24 R60-R62 = SparkFun-Resistors:22OHM: 22Ω resistor; PROD_ID: RES-12427
T1-T3 = transistor:*-NPN_DRIVER-: NPN Bias Resistor Transistor
U1 = TPD4F003DQDR:TPD4F003DQDR; COPYRIGHT: Copyright (C) 2023 Ultra Librarian. All rights reserved.; DIGI-KEY_PART_NUMBER_1: 296-25817-1-ND; DIGI-KEY_PART_NUMBER_2: 296-25817-2-ND; DIGI-KEY_PART_NUMBER_3: 296-25817-6-ND; DIGI-KEY_PART_NUMBER_4: 2156-TPD4F003DQDR-ND; MANUFACTURER_PART_NUMBER: TPD4F003DQDR; MFR_NAME: Texas Instruments
U2-U4 = BMI088:BMI088: High-performance 6-axis inertial sensor (accelerometer + gyroscope) Check prices Check availability; AVAILABILITY: In Stock; CHECK_PRICES: https://www.snapeda.com/parts/BMI088/Bosch+Sensortec/view-part/?ref=eda; DESCRIPTION: Accelerometer, Gyroscope, 6 Axis Sensor I2C, SPI Output; MF: Bosch Sensortec; MP: BMI088; PACKAGE: VFLGA-16 Bosch Sensortec; PRICE: None; PURCHASE-URL: https://www.snapeda.com/api/url_track_click_mouser/?unipart_id=2774026&manufacturer=Bosch Sensortec&part_name=BMI088&search_term=None; SNAPEDA_LINK: https://www.snapeda.com/parts/BMI088/Bosch+Sensortec/view-part/?ref=snap
U5 = STM32H743ZIT6:STM32H743ZIT6: High-performance and DSP with DP-FPU, ARM Cortex-M7 MCU with 2MBytes Flash, 1MB RAM, 400 MHz CPU, Art Accelerator, L1... Check availability; AVAILABILITY: In Stock; CHECK_PRICES: https://www.snapeda.com/parts/STM32H743ZIT6/STMicroelectronics/view-part/?ref=eda; DESCRIPTION: ARM® Cortex®-M7 STM32H7 Microcontroller IC 32-Bit Single-Core 480MHz 2MB (2M x 8) FLASH 144-LQFP (20x20); MF: STMicroelectronics; MP: STM32H743ZIT6; PACKAGE: LQFP-144 STMicroelectronics; PRICE: None; PURCHASE-URL: https://www.snapeda.com/api/url_track_click_mouser/?unipart_id=1041111&manufacturer=STMicroelectronics&part_name=STM32H743ZIT6&search_term=stm32h743; SNAPEDA_LINK: https://www.snapeda.com/parts/STM32H743ZIT6/STMicroelectronics/view-part/?ref=snap; SPICEPREFIX: X
U6 U7 U10 = LIS3MDLTR:LIS3MDLTR: LIS3MDL Series 3 Axis ±2/±8/±12/±16 g 3.6V High Performance Magnetometer LGA-12 Check availability; AVAILABILITY: In Stock; CHECK_PRICES: https://www.snapeda.com/parts/LIS3MDLTR/STMicroelectronics/view-part/?ref=eda; DESCRIPTION: Magnetoresistive Sensor X, Y, Z Axis 12-LGA (2x2); MF: STMicroelectronics; MP: LIS3MDLTR; PACKAGE: VFLGA-12 STMicroelectronics; PRICE: None; PURCHASE-URL: https://www.snapeda.com/api/url_track_click_mouser/?unipart_id=382740&manufacturer=STMicroelectronics&part_name=LIS3MDLTR&search_term=None; SNAPEDA_LINK: https://www.snapeda.com/parts/LIS3MDLTR/STMicroelectronics/view-part/?ref=snap
U$1 = ce-capstone:STPS1L30A
X1 = con-jst2:06FLZ-SM1: CONNECTOR
X3 = con-jst:06FLZ-SM1: CONNECTOR; OC_FARNELL: unknown; OC_NEWARK: unknown
Y1 Y2 = ce-capstone:ABLS-8.000MHZ-B2-T: Crystal 8MHz Â±20ppm (Tol) Â±50ppm (Stability) 18pF FUND 80Ohm 2-Pin HC-49/US SMD T/R; AVAILABILITY: Unavailable; DESCRIPTION: 8MHz ±20ppm Crystal 18pF 80 Ohms HC-49/US; MF: Abracon LLC; MP: ABLS-8.000MHZ-B2; PACKAGE: HC-49/US Abracon LLC; PRICE: None

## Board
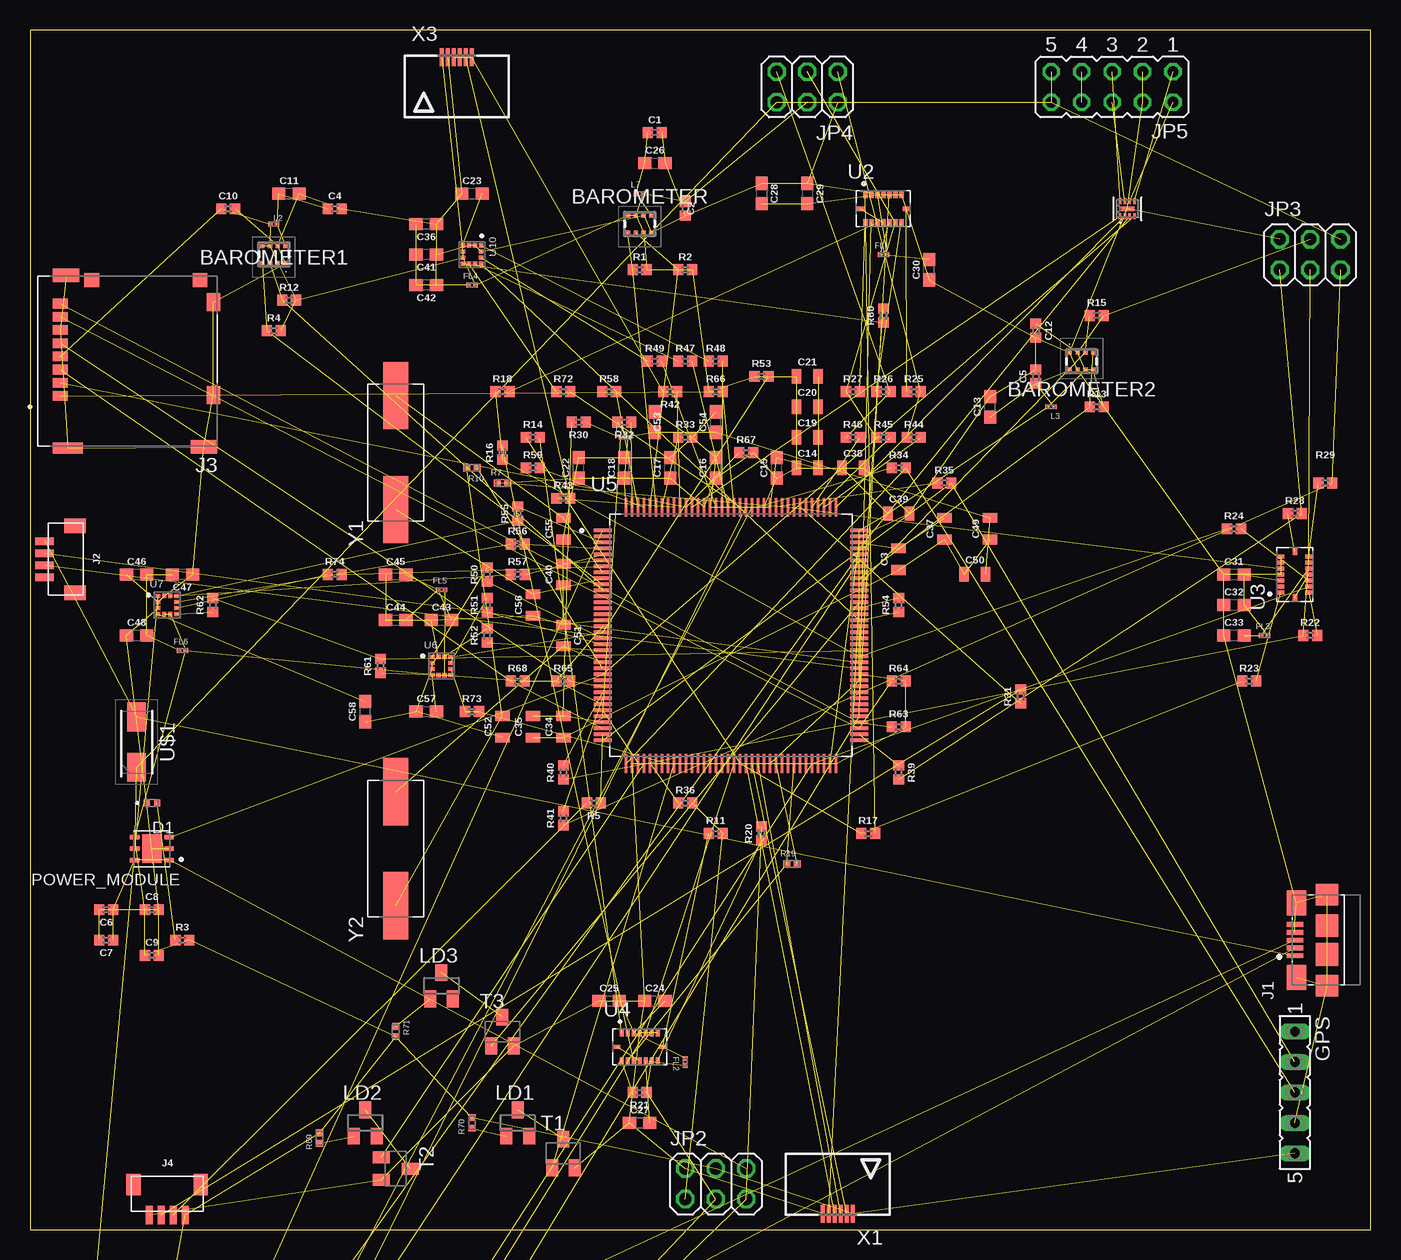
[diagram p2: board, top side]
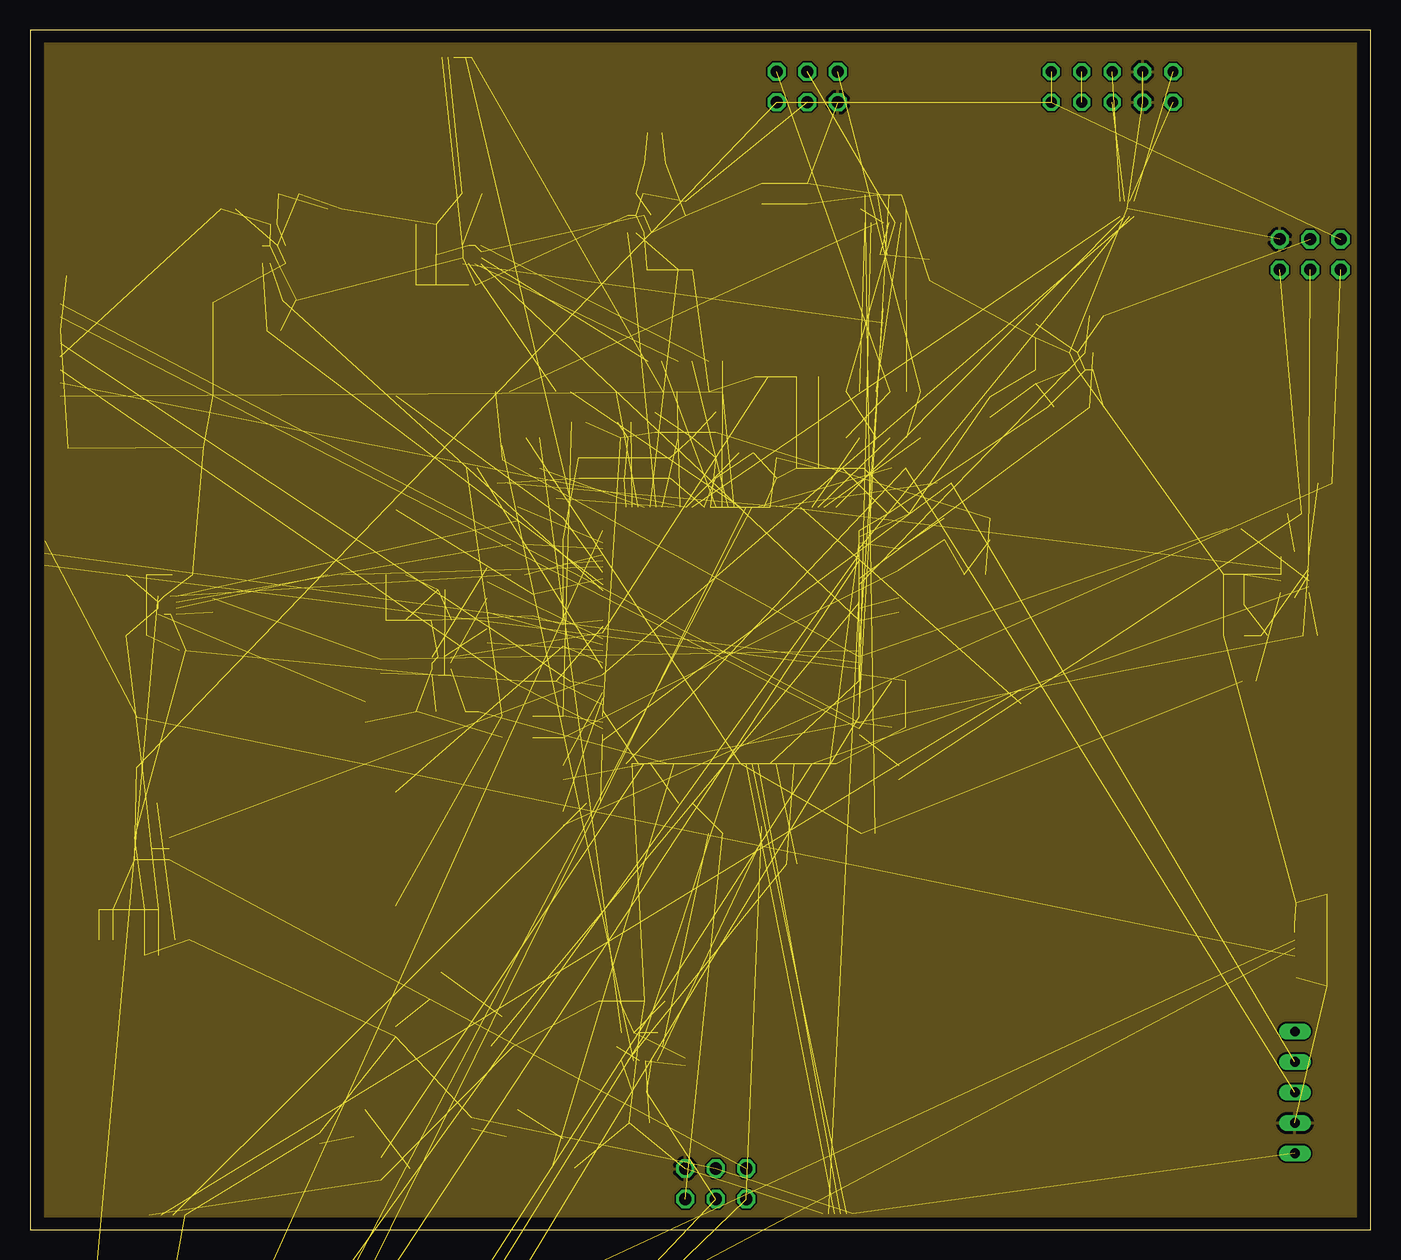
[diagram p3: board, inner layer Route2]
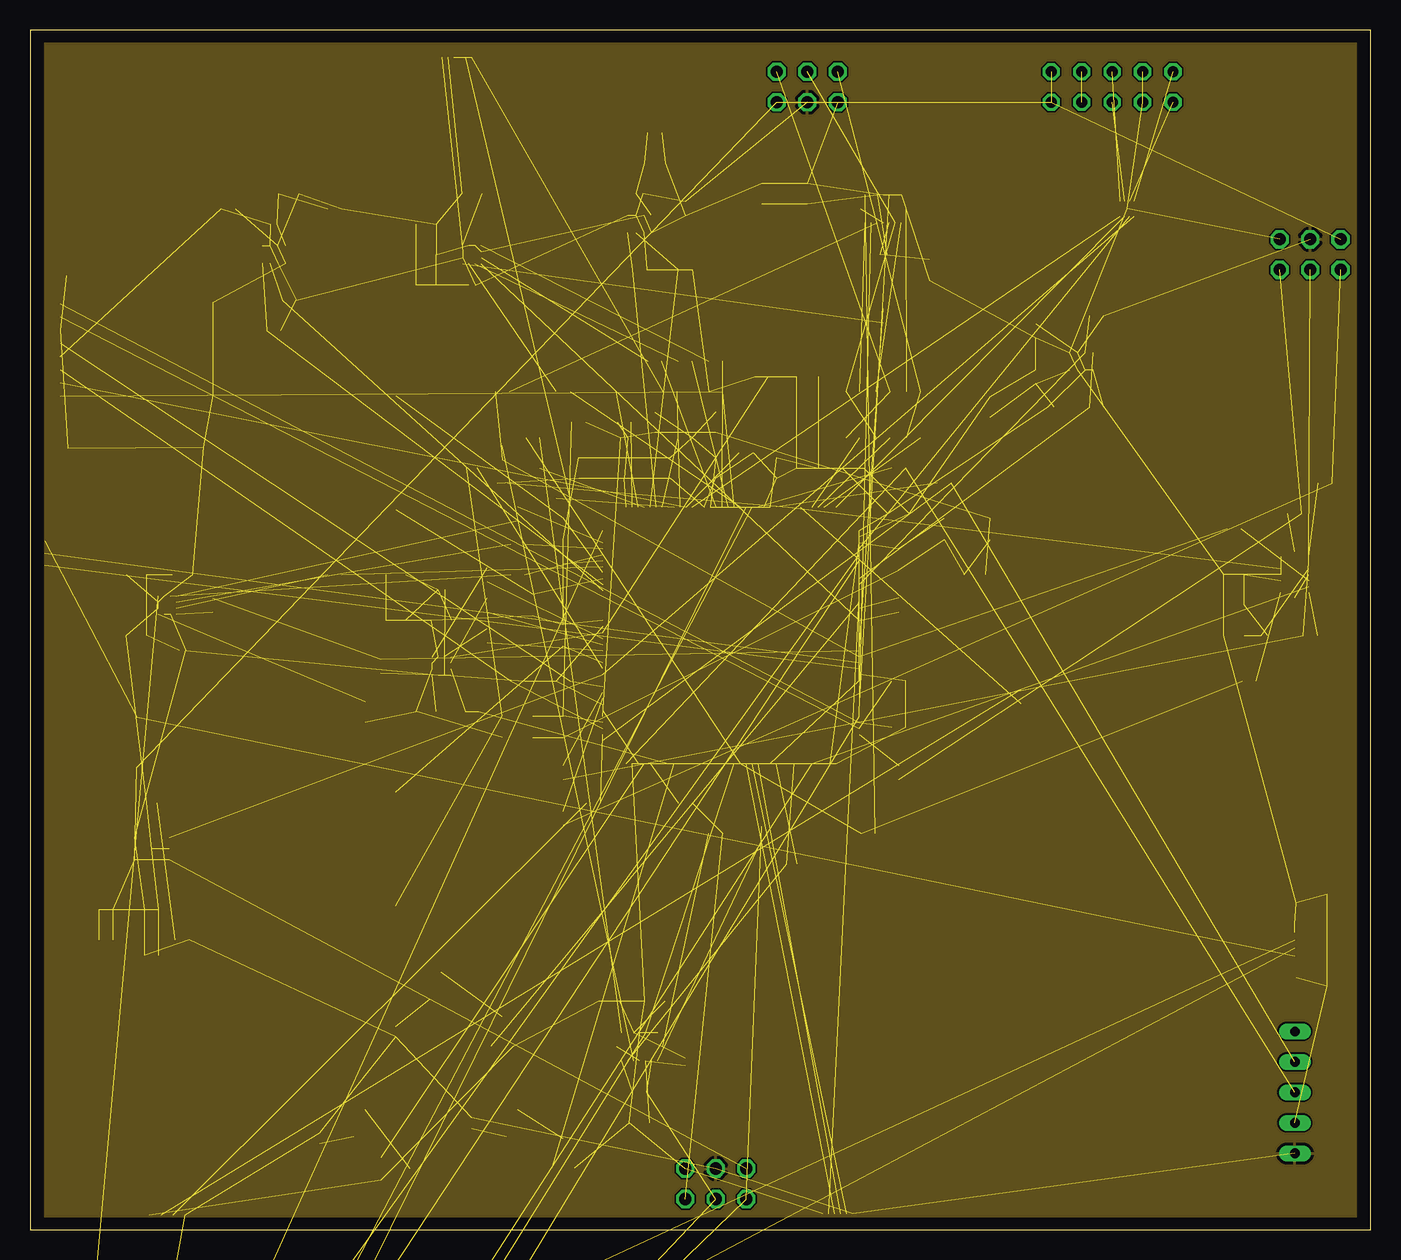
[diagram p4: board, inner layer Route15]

Size 111.74 x 100 mm. Coordinates in mm from the lower left corner, seen from the top.
Outline: 0,0 111.74,0 111.74,100 0,100 0,0
Copper layers (1+2*15+16): Top 0.035mm / dielectric 1.5mm / Route2 0.035mm / dielectric 0.15mm / Route15 0.035mm / dielectric 0.2mm / Bottom 0.035mm
Design rules "default *": minimum track width 6mil, minimum drill 0.35mm, track to track 6mil, track to pad 6mil, pad to pad 6mil, via to via 6mil, smd to smd 6mil, copper to edge 40mil, drill to drill 6mil, minimum pad ring 10mil, minimum via ring 8mil, stop-mask expansion 4mil, vias tented up to drill 0mil, thermal gap 10mil

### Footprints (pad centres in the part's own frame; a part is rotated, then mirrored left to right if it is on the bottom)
DPS310XTSA1 = smd 0.35 x 0.35: 1 0.975,-0.725; 2 0.325,-0.725; 3 -0.325,-0.725; 4 -0.975,-0.725; 5 -0.975,0.725; 6 -0.325,0.725; 7 0.325,0.725; 8 0.975,0.725
0402 = smd 0.85 x 0.9: 1 -0.58,0; 2 0.58,0
0805 = smd 0.8 x 1.2: 1 -0.9,0; 2 0.9,0
0603 = smd 1.1 x 1: 1 -0.85,0; 2 0.85,0
LED_SML-P11UTT86R = smd 0.5 x 0.6: A 0.45,0; C -0.45,0
BEADC0603X33N = smd 0.38 x 0.4: 1 -0.281,0; 2 0.281,0
FE05-1 = drill 0.813 long: 1 -5.08,0; 2 -2.54,0; 3 0,0; 4 2.54,0; 5 5.08,0
AMPHENOL_10118192-0001LF = smd 0.4 x 1.35: 1 -1.3,0; 2 -0.65,0; 3 0,0; 4 0.65,0; 5 1.3,0 | smd 2.1 x 1.6: SH1 -3.1,-0.125; SH2 3.1,-0.125 | smd 1.8 x 1.9: SH3 -3.8,-2.675; SH6 3.8,-2.675 | smd 1.9 x 1.9: SH4 -1.2,-2.675; SH5 1.2,-2.675
BM04B-SRSS-TB = smd 0.6 x 1.55: 1 -1.5,-1.325; 2 -0.5,-1.325; 3 0.5,-1.325; 4 1.5,-1.325 | smd 1.2 x 1.8: M1 -2.8,1.2; M2 2.8,1.2
MOLEX_503182-1852 = smd 0.8 x 1.24: 1 -2.9,6.355; 2 -1.8,6.355; 3 -0.7,6.355; 4 0.4,6.355; 5 1.5,6.355; 6 2.6,6.355; 7 3.7,6.355; 8 4.8,6.355 | smd 1.16 x 1.2: DT 6.74,-5.275 | smd 0.95 x 2.5: P1 -7.245,5.725 | smd 1.15 x 2.2: P2 7.145,5.875; P3 -7.145,-5.605 | smd 1.5 x 1.15: P4 -2.84,-6.4; P5 4.94,-6.4 | smd 1.16 x 1.25: SW 6.74,3.725
2X03 = drill 1.016 octagon: 1 -2.54,-1.27; 2 -2.54,1.27; 3 0,-1.27; 4 0,1.27; 5 2.54,-1.27; 6 2.54,1.27
JP5Q = drill 0.914 octagon: 1 -5.08,-1.27; 2 -5.08,1.27; 3 -2.54,-1.27; 4 -2.54,1.27; 5 0,-1.27; 6 0,1.27; 7 2.54,-1.27; 8 2.54,1.27; 9 5.08,-1.27; 10 5.08,1.27
MICC10 = drill 0.813 long: 1 -5.08,0; 2 5.08,0
SOT23 = smd 1 x 1.4: 1 -0.95,-1.1; 2 0.95,-1.1; 3 0,1.1
SON95P300X300X100-7N = smd 0.84 x 0.4: 1 -1.435,0.95; 2 -1.435,0; 3 -1.435,-0.95; 4 1.435,-0.95; 5 1.435,0; 6 1.435,0.95 | smd 1.625 x 2.365: 7 0,0
RESC1005X35N = smd 0.56 x 0.6: 1 -0.435,0; 2 0.435,0
SC59-BEC = smd 1 x 1.4: B -0.95,-1.2; C 0,1.2; E 0.95,-1.2
DQD8_1P2X0P4 = smd 0.5 x 0.2: 1 -0.625,0.6; 2 -0.625,0.2; 3 -0.625,-0.2; 4 -0.625,-0.6; 5 0.625,-0.6; 6 0.625,-0.2; 7 0.625,0.2; 8 0.625,0.6 | smd 0.4 x 1.2: 9 0,0
PQFN50P450X300X100-16N = smd 0.35 x 0.59: 1 -1.5,1.165; 2 -1,1.165; 3 -0.5,1.165; 4 0,1.165; 5 0.5,1.165; 6 1,1.165; 7 1.5,1.165; 9 1.5,-1.165; 10 1,-1.165; 11 0.5,-1.165; 12 0,-1.165; 13 -0.5,-1.165; 14 -1,-1.165; 15 -1.5,-1.165 | smd 0.59 x 0.35: 8 1.915,0; 16 -1.915,0
QFP50P2200X2200X160-144N = smd 1.56 x 0.28: 1 -10.68,8.75; 2 -10.68,8.25; 3 -10.68,7.75; 4 -10.68,7.25; 5 -10.68,6.75; 6 -10.68,6.25; 7 -10.68,5.75; 8 -10.68,5.25; 9 -10.68,4.75; 10 -10.68,4.25; 11 -10.68,3.75; 12 -10.68,3.25; 13 -10.68,2.75; 14 -10.68,2.25; 15 -10.68,1.75; 16 -10.68,1.25; 17 -10.68,0.75; 18 -10.68,0.25; 19 -10.68,-0.25; 20 -10.68,-0.75; 21 -10.68,-1.25; 22 -10.68,-1.75; 23 -10.68,-2.25; 24 -10.68,-2.75; 25 -10.68,-3.25; 26 -10.68,-3.75; 27 -10.68,-4.25; 28 -10.68,-4.75; 29 -10.68,-5.25; 30 -10.68,-5.75; 31 -10.68,-6.25; 32 -10.68,-6.75; 33 -10.68,-7.25; 34 -10.68,-7.75; 35 -10.68,-8.25; 36 -10.68,-8.75; 73 10.68,-8.75; 74 10.68,-8.25; 75 10.68,-7.75; 76 10.68,-7.25; 77 10.68,-6.75; 78 10.68,-6.25; 79 10.68,-5.75; 80 10.68,-5.25; 81 10.68,-4.75; 82 10.68,-4.25; 83 10.68,-3.75; 84 10.68,-3.25; 85 10.68,-2.75; 86 10.68,-2.25; 87 10.68,-1.75; 88 10.68,-1.25; 89 10.68,-0.75; 90 10.68,-0.25; 91 10.68,0.25; 92 10.68,0.75; 93 10.68,1.25; 94 10.68,1.75; 95 10.68,2.25; 96 10.68,2.75; 97 10.68,3.25; 98 10.68,3.75; 99 10.68,4.25; 100 10.68,4.75; 101 10.68,5.25; 102 10.68,5.75; 103 10.68,6.25; 104 10.68,6.75; 105 10.68,7.25; 106 10.68,7.75; 107 10.68,8.25; 108 10.68,8.75 | smd 0.28 x 1.56: 37 -8.75,-10.68; 38 -8.25,-10.68; 39 -7.75,-10.68; 40 -7.25,-10.68; 41 -6.75,-10.68; 42 -6.25,-10.68; 43 -5.75,-10.68; 44 -5.25,-10.68; 45 -4.75,-10.68; 46 -4.25,-10.68; 47 -3.75,-10.68; 48 -3.25,-10.68; 49 -2.75,-10.68; 50 -2.25,-10.68; 51 -1.75,-10.68; 52 -1.25,-10.68; 53 -0.75,-10.68; 54 -0.25,-10.68; 55 0.25,-10.68; 56 0.75,-10.68; 57 1.25,-10.68; 58 1.75,-10.68; 59 2.25,-10.68; 60 2.75,-10.68; 61 3.25,-10.68; 62 3.75,-10.68; 63 4.25,-10.68; 64 4.75,-10.68; 65 5.25,-10.68; 66 5.75,-10.68; 67 6.25,-10.68; 68 6.75,-10.68; 69 7.25,-10.68; 70 7.75,-10.68; 71 8.25,-10.68; 72 8.75,-10.68; 109 8.75,10.68; 110 8.25,10.68; 111 7.75,10.68; 112 7.25,10.68; 113 6.75,10.68; 114 6.25,10.68; 115 5.75,10.68; 116 5.25,10.68; 117 4.75,10.68; 118 4.25,10.68; 119 3.75,10.68; 120 3.25,10.68; 121 2.75,10.68; 122 2.25,10.68; 123 1.75,10.68; 124 1.25,10.68; 125 0.75,10.68; 126 0.25,10.68; 127 -0.25,10.68; 128 -0.75,10.68; 129 -1.25,10.68; 130 -1.75,10.68; 131 -2.25,10.68; 132 -2.75,10.68; 133 -3.25,10.68; 134 -3.75,10.68; 135 -4.25,10.68; 136 -4.75,10.68; 137 -5.25,10.68; 138 -5.75,10.68; 139 -6.25,10.68; 140 -6.75,10.68; 141 -7.25,10.68; 142 -7.75,10.68; 143 -8.25,10.68; 144 -8.75,10.68
XDCR_LIS3MDLTR = smd 0.375 x 0.35: 1 -0.762,0.75; 2 -0.762,0.25; 3 -0.762,-0.25; 4 -0.762,-0.75; 7 0.762,-0.75; 8 0.762,-0.25; 9 0.762,0.25; 10 0.762,0.75 | smd 0.35 x 0.375: 5 -0.25,-0.762; 6 0.25,-0.762; 11 0.25,0.762; 12 -0.25,0.762
DIOM5226X223N = smd 2.4 x 1.55: 1 -2.1,0; 2 2.1,0
6FLZ-SM = smd 0.3 x 1.5: 1 -1.25,2.5; 2 -0.75,2.5; 3 -0.25,2.5; 4 0.25,2.5; 5 0.75,2.5; 6 1.25,2.5
XTAL_ABLS-8.000MHZ-B2-T = smd 5.6 x 2.1: 1 -4.75,0; 2 4.75,0

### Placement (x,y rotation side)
BAROMETER  50.8,83.82 0 top
BAROMETER1  20.32,81.28 0 top
BAROMETER2  87.63,72.39 180 top
C1  52.07,91.44 0 top
C2  54.61,85.09 270 top
C3  72.39,55.88 90 top
C4  25.4,85.09 0 top
C5  83.82,71.12 90 top
C6  6.35,26.67 180 top
C7  6.35,24.13 180 top
C8  10.16,26.67 0 top
C9  10.16,22.86 0 top
C10  16.51,85.09 0 top
C11  21.59,86.36 0 top
C12  83.82,74.93 270 top
C13  80.01,68.58 90 top
C14  64.77,63.5 0 top
C15  62.23,63.5 90 top
C16  57.15,63.5 90 top
C17  53.34,63.5 90 top
C18  49.53,63.5 90 top
C19  64.77,66.04 0 top
C20  64.77,68.58 0 top
C21  64.77,71.12 0 top
C22  45.72,63.5 90 top
C23  36.83,86.36 0 top
C24  52.07,19.05 0 top
C25  48.26,19.05 0 top
C26  52.07,88.9 0 top
C27  50.8,8.89 0 top
C28  60.96,86.36 270 top
C29  64.77,86.36 270 top
C30  74.93,80.01 90 top
C31  100.33,54.61 0 top
C32  100.33,52.07 0 top
C33  100.33,49.53 0 top
C34  44.45,41.91 90 top
C35  41.91,41.91 90 top
C36  33.02,83.82 180 top
C37  76.2,58.42 90 top
C38  68.58,63.5 0 top
C39  72.39,59.69 0 top
C40  44.45,54.61 90 top
C41  33.02,81.28 180 top
C42  33.02,78.74 180 top
C43  34.29,50.8 0 top
C44  30.48,50.8 0 top
C45  30.48,54.61 0 top
C46  8.89,54.61 0 top
C47  12.7,54.61 180 top
C48  8.89,49.53 0 top
C49  80.01,58.42 90 top
C50  78.74,54.61 0 top
C51  44.45,49.53 270 top
C52  39.37,41.91 90 top
C53  52.07,67.31 90 top
C54  57.15,67.31 90 top
C55  44.45,58.42 90 top
C56  41.91,52.07 90 top
C57  33.02,43.18 0 top
C58  27.94,43.18 90 top
C59  not placed on the board
C60  not placed on the board
D1  10.16,35.56 0 top
FL1  71.12,81.28 0 top
FL2  54.61,13.97 90 top
FL3  102.87,49.53 0 top
FL4  36.83,78.74 0 top
FL5  34.29,53.34 0 top
FL6  12.7,48.26 0 top
GPS  105.41,11.43 270 top
J1  105.41,24.13 90 top
J2  2.54,55.88 270 top
J3  8.89,72.39 90 top
J4  11.43,2.54 0 top
JP2  57.15,3.81 0 top
JP3  106.68,81.28 0 top
JP4  64.77,95.25 180 top
JP5  90.17,95.25 180 top
L1  49.53,66.04 0 top
L2  20.32,83.82 180 top
L3  85.09,68.58 180 top
L6  not placed on the board
L7  50.8,86.36 0 top
L8  not placed on the board
LD1  40.64,8.89 0 top
LD2  27.94,8.89 0 top
LD3  34.29,20.32 0 top
POWER_MODULE  10.16,31.75 180 top
R1  50.8,80.01 0 top
R2  54.61,80.01 0 top
R3  12.7,24.13 0 top
R4  20.32,74.93 0 top
R5  46.99,35.56 180 top
R6  not placed on the board
R7  39.37,62.23 0 top
R8  not placed on the board
R9  not placed on the board
R10  36.83,63.5 180 top
R11  57.15,33.02 0 top
R12  21.59,77.47 0 top
R13  88.9,68.58 0 top
R14  41.91,66.04 0 top
R15  88.9,76.2 0 top
R16  39.37,64.77 90 top
R17  69.85,33.02 0 top
R18  39.37,69.85 0 top
R19  63.5,30.48 0 top
R20  60.96,33.02 90 top
R21  50.8,11.43 180 top
R22  106.68,49.53 0 top
R23  101.6,45.72 0 top
R24  100.33,58.42 0 top
R25  73.66,69.85 0 top
R26  71.12,69.85 0 top
R27  68.58,69.85 0 top
R28  105.41,59.69 0 top
R29  107.95,62.23 0 top
R30  45.72,67.31 180 top
R31  82.55,44.45 90 top
R32  49.53,67.31 180 top
R33  54.61,66.04 0 top
R34  72.39,63.5 0 top
R35  76.2,62.23 0 top
R36  54.61,35.56 0 top
R39  72.39,38.1 270 top
R40  44.45,38.1 90 top
R41  44.45,34.29 90 top
R42  53.34,69.85 180 top
R43  44.45,60.96 0 top
R44  73.66,66.04 0 top
R45  71.12,66.04 0 top
R46  68.58,66.04 0 top
R47  54.61,72.39 0 top
R48  57.15,72.39 0 top
R49  52.07,72.39 0 top
R50  38.1,54.61 90 top
R51  38.1,52.07 90 top
R52  38.1,49.53 90 top
R53  60.96,71.12 0 top
R54  72.39,52.07 90 top
R55  40.64,59.69 90 top
R56  40.64,57.15 0 top
R57  40.64,54.61 0 top
R58  48.26,69.85 0 top
R59  41.91,63.5 0 top
R60  71.12,76.2 90 top
R61  29.21,46.99 90 top
R62  15.24,52.07 90 top
R63  72.39,41.91 0 top
R64  72.39,45.72 0 top
R65  44.45,45.72 0 top
R66  57.15,69.85 0 top
R67  59.69,64.77 0 top
R68  40.64,45.72 0 top
R69  24.13,7.62 90 top
R70  36.83,8.89 90 top
R71  30.48,16.51 270 top
R72  44.45,69.85 0 top
R73  36.83,43.18 0 top
R74  25.4,54.61 0 top
R75  not placed on the board
R76  not placed on the board
R77  not placed on the board
T1  44.45,6.35 0 top
T2  30.48,5.08 270 top
T3  39.37,16.51 0 top
U1  91.44,85.09 90 top
U2  71.12,85.09 0 top
U3  105.41,54.61 90 top
U4  50.8,15.24 0 top
U5  58.42,49.53 0 top
U6  34.29,46.99 0 top
U7  11.43,52.07 0 top
U10  36.83,81.28 270 top
U$1  8.89,40.64 90 top
X1  67.31,3.81 180 top
X3  35.56,95.25 0 top
Y1  30.48,64.77 90 top
Y2  30.48,31.75 90 top

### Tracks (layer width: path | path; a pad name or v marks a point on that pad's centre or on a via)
3.3V  (1 unrouted)
3V2  (3 unrouted)
3V3  (83 unrouted)
  pour Route15: 1.27,0 1.27,99.06 110.49,99.06 110.49,0
3V4  (3 unrouted)
3V5  (3 unrouted)
5V  (9 unrouted)
5V_IN  (2 unrouted)
AGND  (5 unrouted)
CSB_ACCEL1  (2 unrouted)
CSB_ACCEL2  (2 unrouted)
CSB_ACCEL3  (2 unrouted)
CSB_GYRO1  (2 unrouted)
CSB_GYRO2  (2 unrouted)
CSB_GYRO3  (1 unrouted)
DM  (2 unrouted)
DP  (2 unrouted)
DRDY1  (1 unrouted)
DRDY2  (3 unrouted)
DRDY3  (1 unrouted)
EXTI0  (1 unrouted)
EXTI0_1  (1 unrouted)
EXTI0_2  (1 unrouted)
EXTI2  (1 unrouted)
EXTI2_1  (1 unrouted)
EXTI2_2  (1 unrouted)
GND  (115 unrouted)
  pour Route2: 1.27,0 1.27,99.06 110.49,99.06 110.49,0
GPIO1  (1 unrouted)
GPIO_EXTI0  (3 unrouted)
GPIO_EXTI2  (3 unrouted)
GPIO_EXTI3  (3 unrouted)
I2C1_SCL  (2 unrouted)
I2C1_SDA  (2 unrouted)
I2C2_SCL  (2 unrouted)
I2C2_SDA  (2 unrouted)
I2C3_SCL  (2 unrouted)
I2C3_SDA  (2 unrouted)
INT1  (1 unrouted)
LED01  (1 unrouted)
LED02  (1 unrouted)
LED03  (1 unrouted)
N$1  (1 unrouted)
N$2  (3 unrouted)
N$3  (3 unrouted)
N$4  (1 unrouted)
N$5  (1 unrouted)
N$6  (3 unrouted)
N$7  (2 unrouted)
N$8  (2 unrouted)
N$9  (2 unrouted)
N$10  (2 unrouted)
N$11  (1 unrouted)
N$12  (1 unrouted)
N$13  (1 unrouted)
N$14  (1 unrouted)
N$16  (3 unrouted)
N$17  (1 unrouted)
N$18  (1 unrouted)
N$20  (1 unrouted)
N$21  (1 unrouted)
N$22  (1 unrouted)
N$23  (1 unrouted)
N$24  (1 unrouted)
N$25  (1 unrouted)
N$26  (1 unrouted)
N$27  (1 unrouted)
N$28  (1 unrouted)
N$29  (1 unrouted)
N$30  (1 unrouted)
N$31  (1 unrouted)
N$32  (1 unrouted)
N$33  (1 unrouted)
N$36  (1 unrouted)
N$37  (1 unrouted)
N$38  (1 unrouted)
N$39  (1 unrouted)
N$40  (1 unrouted)
N$41  (1 unrouted)
N$42  (1 unrouted)
N$43  (1 unrouted)
N$44  (1 unrouted)
N$45  (1 unrouted)
N$46  (1 unrouted)
N$47  (1 unrouted)
N$48  (1 unrouted)
N$49  (1 unrouted)
N$50  (1 unrouted)
N$51  (1 unrouted)
N$52  (1 unrouted)
N$53  (3 unrouted)
N$54  (1 unrouted)
N$55  (3 unrouted)
N$56  (1 unrouted)
N$57  (1 unrouted)
N$58  (1 unrouted)
N$59  (1 unrouted)
N$60  (1 unrouted)
N$61  (1 unrouted)
N$62  (1 unrouted)
N$63  (1 unrouted)
N$64  (1 unrouted)
N$65  (1 unrouted)
N$66  (1 unrouted)
N$67  (1 unrouted)
N$68  (1 unrouted)
N$69  (1 unrouted)
NRST  (2 unrouted)
NRST_O  (1 unrouted)
OSC32_IN  (2 unrouted)
OSC32_OUT  (2 unrouted)
OSC_IN  (2 unrouted)
OSC_OUT  (1 unrouted)
SDMCC_CK  (2 unrouted)
SDMCC_CMD  (2 unrouted)
SDMCC_D0  (2 unrouted)
SDMCC_D1  (2 unrouted)
SDMCC_D2  (2 unrouted)
SDMCC_D3  (2 unrouted)
SPI1_MISO  (3 unrouted)
SPI1_MOSI  (2 unrouted)
SPI1_SCK  (2 unrouted)
SPI2_MISO  (3 unrouted)
SPI2_MOSI  (2 unrouted)
SPI2_SCK  (2 unrouted)
SPI3_MISO  (3 unrouted)
SPI3_MOSI  (2 unrouted)
SPI3_SCK  (2 unrouted)
SPI4_CS  (1 unrouted)
SPI4_MISO  (1 unrouted)
SPI4_MOSI  (1 unrouted)
SPI4_SCK  (1 unrouted)
SPI5_CS  (2 unrouted)
SPI5_MISO  (1 unrouted)
SPI5_MOSI  (1 unrouted)
SPI5_SCK  (1 unrouted)
SPI6_CS  (2 unrouted)
SPI6_MISO  (1 unrouted)
SPI6_MOSI  (1 unrouted)
SPI6_SCK  (1 unrouted)
SWCLK  (1 unrouted)
SWCLK_O  (1 unrouted)
SWDIO  (1 unrouted)
SWDIO_O  (1 unrouted)
SWO  (1 unrouted)
SWO_O  (1 unrouted)
UART4_RX  (1 unrouted)
UART4_TX  (1 unrouted)
UART5_RX  (2 unrouted)
UART5_TX  (1 unrouted)
UART7_RX  (1 unrouted)
UART7_TX  (1 unrouted)
UART8_CTS  (1 unrouted)
UART8_RTS  (1 unrouted)
USART2_RX  (2 unrouted)
USART2_TX  (2 unrouted)
USB_FS_DM  (2 unrouted)
USB_FS_DP  (2 unrouted)
VBAT  (1 unrouted)
VCAP  (3 unrouted)
VDDA  (3 unrouted)
VREFP  (6 unrouted)
XSHUT  (1 unrouted)

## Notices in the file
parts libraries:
SparkFun-Capacitors: Licensing: Creative Commons ShareAlike 4.0 International - https://creativecommons.org/licenses/by-sa/4.0
